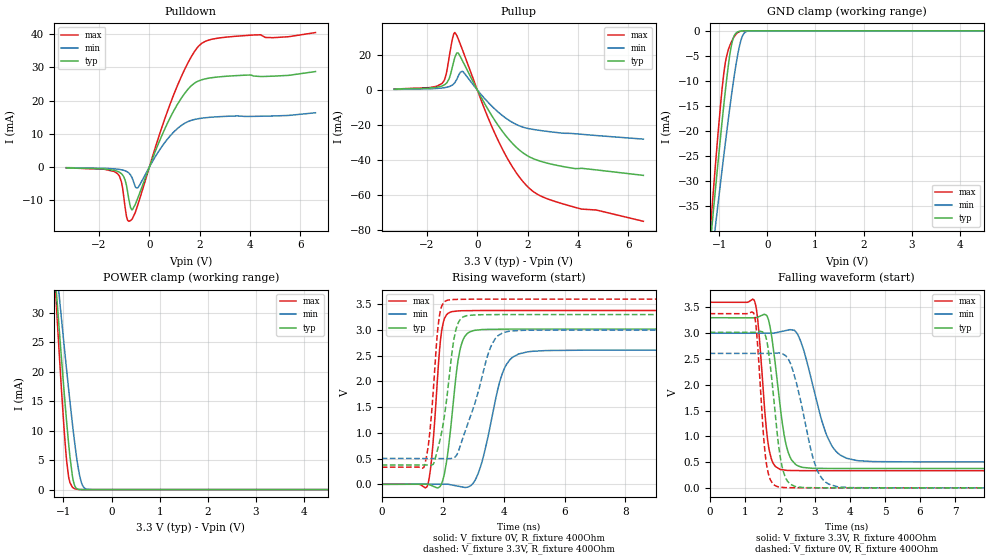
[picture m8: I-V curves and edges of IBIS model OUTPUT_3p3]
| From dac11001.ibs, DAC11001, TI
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|   OUTPUT_3p3 Model
[Model]   OUTPUT_3p3
Model_type   3-state
Polarity   Non-Inverting
Vmeas = 1.65
Vref = 0
Cref = 2pF
Rref = 100000
|   typ   min   max
C_comp   1.526pF   1.485pF   1.555pF
[Voltage Range]   3.3   3   3.6
[Temperature Range]   25   125   -40
[Pullup Reference]   3.3   3   3.6
[Pulldown Reference]   0   0   0
[Power Clamp Reference]   3.3   3   3.6
[GND Clamp Reference]   0   0   0
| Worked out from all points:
|   slope of the pulldown table from 0 to 0.495 V, typ, clamps not added: 52.4 ohm
|   slope of the pullup table from 0 to 0.495 V, typ, clamps not added: 38.7 ohm
|   GND clamp passes 1 mA (typ) near -0.69 V on its own axis
|   POWER clamp passes 1 mA (typ) near -0.78 V on its own axis
|   falling waveform, V_fixture 3.3V, R_fixture 400Ohm: 20-80 % time 330ps typ, 597ps min, 231ps max; typ from 3.3 V to 0.375 V
|   rising waveform, V_fixture 0V, R_fixture 400Ohm: 20-80 % time 341ps typ, 591ps min, 247ps max; typ from 0 V to 3.02 V
|   rising waveform, V_fixture 3.3V, R_fixture 400Ohm: 20-80 % time 393ps typ, 753ps min, 254ps max; typ from 0.375 V to 3.3 V
|   falling waveform, V_fixture 0V, R_fixture 400Ohm: 20-80 % time 290ps typ, 519ps min, 206ps max; typ from 3.02 V to 0 V
[Pulldown]
|   Voltage   I(typ)   I(min)   I(max)
-3.3V     -212.9uA   -153.4uA   -219.2uA
-1.28V    -1.217mA   -601.6uA   -1.866mA
-1.112V   -1.958mA   -795uA     -4.347mA
-973.5mV  -3.674mA   -1.076mA   -11.5mA
-864.6mV  -7.371mA   -1.475mA   -15.98mA
-745.8mV  -12.22mA   -2.368mA   -16.08mA
-468.6mV  -9.503mA   -6.301mA   -11.59mA
848.1mV   15.18mA    9.584mA    19.43mA
1.403V    22.16mA    13.18mA    29.38mA
1.957V    25.94mA    14.58mA    36.4mA
2.927V    27.26mA    15.23mA    39mA
6.6V      28.75mA    16.35mA    40.49mA
[GND Clamp]
|   Voltage   I(typ)   I(min)   I(max)
-3.3V     -270mA     -231.5mA   -318.5mA
-1.211V   -45.1mA    -49.98mA   -42.91mA
-1.112V   -34.95mA   -41.72mA   -30.68mA
-1.073V   -30.95mA   -38.44mA   -25.93mA
-963.6mV  -20.24mA   -29.56mA   -13.77mA
-884.4mV  -12.92mA   -23.26mA   -7.01mA
-815.1mV  -7.187mA   -17.92mA   -3.873mA
-745.8mV  -2.848mA   -12.85mA   -2.186mA
-617.1mV  -220.8uA   -4.82mA    -373.5uA
-508.2mV  -17.82uA   -844.2uA   -28.78uA
-379.5mV  -412.4nA   -27.33uA   -420.9nA
6.6V      0A         0A         0A
[Pullup]
|   Voltage   I(typ)   I(min)   I(max)
-3.3V     402.4uA    279.4uA    471.1uA
-1.399V   2.244mA    1.086mA    3.724mA
-1.231V   3.741mA    1.458mA    9.154mA
-1.122V   6.261mA    1.866mA    18.16mA
-983.4mV  13.43mA    2.843mA    29.35mA
-884.4mV  18.85mA    4.292mA    32.78mA
-755.7mV  21.09mA    7.88mA     29.2mA
-577.5mV  16.38mA    10.51mA    22.5mA
848.1mV   -20.69mA   -12.9mA    -29.5mA
1.957V    -37.39mA   -21.9mA    -54.74mA
3.204V    -43.3mA    -24.47mA   -64.36mA
6.6V      -48.92mA   -28.17mA   -75.2mA
[POWER Clamp]
|   Voltage   I(typ)   I(min)   I(max)
-3.3V     283.1mA    229.6mA    356.1mA
-1.191V   38.42mA    41.64mA    37.54mA
-1.142V   33.01mA    37.43mA    30.56mA
-1.082V   26.61mA    32.44mA    22.41mA
-993.3mV  17.34mA    25.09mA    11.05mA
-933.9mV  11.54mA    20.31mA    4.906mA
-864.6mV  5.579mA    14.94mA    1.195mA
-815.1mV  2.393mA    11.29mA    425.4uA
-765.6mV  672.5uA    7.903mA    151.1uA
-636.9mV  10.62uA    1.492mA    6.782uA
-508.2mV  197.1nA    57.28uA    101.5nA
6.6V      0A         0A         0A
[Ramp]
R_load = 400
|   typ   min   max
dV/dt_r   1.81066/3.40438e-10   1.56477/5.91388e-10   2.02742/2.46568e-10
dV/dt_f   1.75528/3.28367e-10   1.49814/5.95526e-10   1.96053/2.30287e-10
[Falling Waveform]
V_fixture = 3.3V
V_fixture_min = 3V
V_fixture_max = 3.6V
R_fixture = 400Ohm
C_fixture = 0F
|   Time   V(typ)   V(min)   V(max)
0s        3.3V       3V         3.6V
1.276ns   3.299V     2.999V     3.63V
1.397ns   3.319V     2.999V     3.071V
1.629ns   3.339V     2.999V     1.069V
1.809ns   2.737V     2.999V     480.9mV
2.217ns   739.6mV    3.058V     337.6mV
2.786ns   388.3mV    2.412V     332.7mV
3.625ns   374.8mV    693.5mV    332.7mV
5.878ns   374.8mV    503.3mV    332.7mV
3.5us     374.5mV    503.1mV    332.5mV
[Rising Waveform]
V_fixture = 0V
V_fixture_min = 0V
V_fixture_max = 0V
R_fixture = 400Ohm
C_fixture = 0F
|   Time   V(typ)   V(min)   V(max)
0s        2.425nV    -6.045nV   2.256nV
1.497ns   1.201mV    885.3uV    -32.03mV
1.659ns   -30.29mV   981.1uV    631.5mV
1.923ns   -34.23mV   1.137mV    2.765V
2.152ns   538.2mV    1.273mV    3.311V
2.598ns   2.684V     -46.93mV   3.374V
3.249ns   3.005V     351.8mV    3.379V
4.192ns   3.017V     2.411V     3.379V
6.67ns    3.017V     2.608V     3.379V
3.5us     3.018V     2.608V     3.379V
[Rising Waveform]
V_fixture = 3.3V
V_fixture_min = 3V
V_fixture_max = 3.6V
R_fixture = 400Ohm
C_fixture = 0F
|   Time   V(typ)   V(min)   V(max)
0s        374.5mV    503.1mV    332.5mV
1.38ns    375.9mV    501.1mV    327.2mV
1.698ns   398.6mV    500.7mV    1.87V
1.844ns   700.5mV    500.5mV    3.046V
1.984ns   1.067V     500.3mV    3.485V
2.448ns   3.034V     559.7mV    3.595V
3.04ns    3.291V     1.54V      3.6V
3.816ns   3.299V     2.889V     3.6V
5.878ns   3.3V       3V         3.6V
3.5us     3.3V       3V         3.6V
[Falling Waveform]
|Gnd
V_fixture = 0V
V_fixture_min = 0V
V_fixture_max = 0V
R_fixture = 400Ohm
C_fixture = 0F
|   Time   V(typ)   V(min)   V(max)
0s        3.018V     2.608V     3.379V
1.256ns   3.017V     2.607V     3.387V
1.349ns   3.025V     2.607V     2.932V
1.57ns    2.985V     2.607V     743.7mV
1.729ns   2.374V     2.607V     160.7mV
2.097ns   327.5mV    2.592V     7.553mV
2.713ns   4.726mV    1.302V     249.7uV
3.302ns   421.1uV    113.7mV    249.6uV
4.926ns   286.1uV    306.4uV    249.5uV
3.5us     -23.99nV   -54.56nV   -151.8nV
